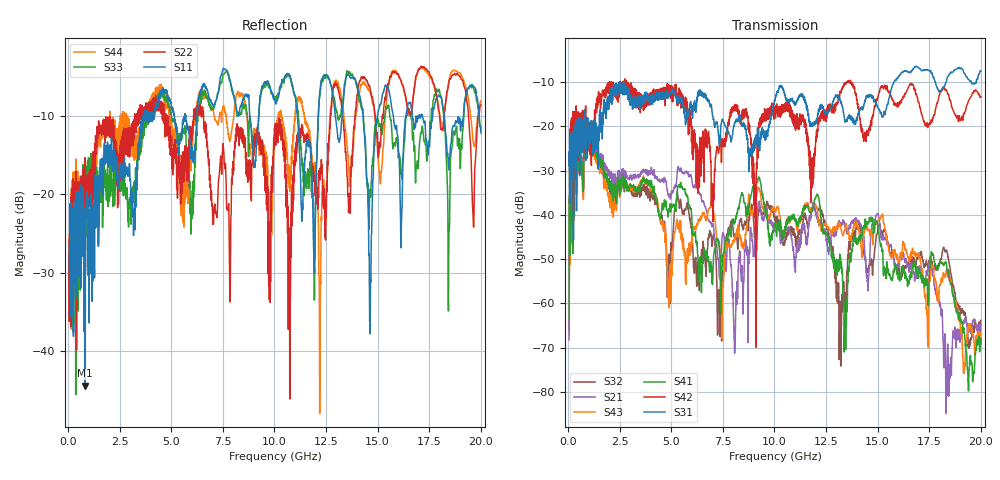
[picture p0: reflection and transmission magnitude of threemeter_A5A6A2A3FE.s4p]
! FILE: D:\iPass\iPassCable1005\iPassCable\SOLT_cal\threemeter_A5A6A2A3FE.s4p
# MHz S MA R 50.00
! FREQ  S11  S12  S13  S14
!  S21  S22  S23  S24
!  S31  S32  S33  S34
!  S41  S42  S43  S44
!  MAG  ANG  MAG  ANG  MAG  ANG  MAG  ANG
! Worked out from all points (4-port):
!   1996 points, 50 MHz to 20 GHz, reference 50 ohm
!   strongest paths, dB at 50 MHz, 5.04 GHz, 10.03 GHz, 15.02 GHz, 20 GHz:
!     S31: -29.0, -11.9, -13.8, -15.9, -7.5
!     S42: -27.3, -12.2, -15.4, -13.2, -13.3
!     S41: -63.7, -38.3, -42.7, -43.2, -69.3
!     S43: -61.9, -51.9, -39.3, -41.2, -67.3
!     S21: -68.3, -35.1, -42.8, -39.9, -64.8
!     S32: -65.8, -47.4, -40.7, -42.7, -63.9
!   lowest |S11| = -44.4 dB at 830 MHz (marker M1), VSWR 1.01, Z = 50.3 - j0.541 ohm
!   |S11| at or under -10 dB: start of sweep to 3.653 GHz; 11.11 GHz to 12.12 GHz (1.013 GHz wide, 8.72 % of centre); 18.22 GHz to 19.16 GHz (933.2 MHz wide, 4.99 % of centre)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
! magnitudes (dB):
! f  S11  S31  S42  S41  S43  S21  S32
! 50 MHz  -26.7  -29.0  -27.3  -63.7  -61.9  -68.3  -65.8
! 830 MHz  -44.4  -19.2  -17.5  -27.0  -27.7  -26.0  -27.3
! 8.08 GHz  -7.9  -19.1  -16.0  -41.8  -45.6  -69.8  -44.5
! 11.89 GHz  -24.9  -19.1  -31.8  -38.0  -37.9  -37.1  -37.5
! 13.21 GHz  -12.2  -14.7  -12.2  -50.6  -43.0  -42.0  -74.2
! 14.05 GHz  -6.6  -17.1  -16.0  -45.4  -42.9  -41.6  -41.6
! 20 GHz  -12.2  -7.5  -13.3  -69.3  -67.3  -64.8  -63.9
